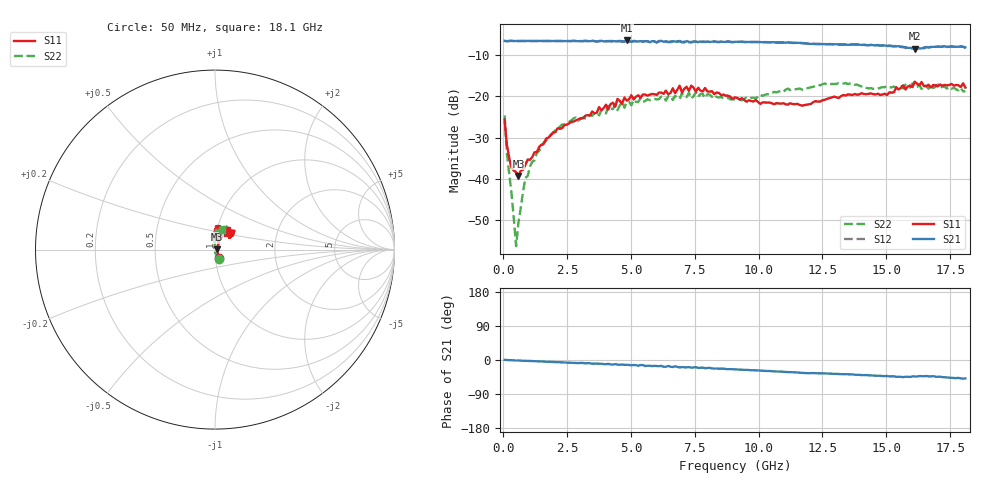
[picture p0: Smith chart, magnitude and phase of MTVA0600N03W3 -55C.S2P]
! Network Analyzer HP8720D.06.14 Serial No. US36140669
!  8 Jul 2005  09:57:14
! Frequency  S11  S21  S12  S22
# HZ  S  DB R 50
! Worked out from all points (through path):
!   201 points, 50 MHz to 18.1 GHz, reference 50 ohm
!   highest |S21| = -6.50 dB at 4.833 GHz (marker M1); lowest = -8.5 dB at 16.11 GHz (marker M2)
!   group delay of S21, straight-line fit = 7.68 ps
!   lowest |S11| = -39.2 dB at 591.5 MHz (marker M3), VSWR 1.02, Z = 51.1 + j0.0803 ohm
!   |S11| at or under -10 dB: start of sweep to end of sweep
!   |S22| runs from -56.3 to -16.8 dB; largest |S21 - S12| = 0.017
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5e7  -25.71 -67.1  -6.58 0.4  -6.62 0.3  -24.64 -67.0
1.4025e8  -31.84 -52.1  -6.69 -0.1  -6.68 -0.2  -33.88 -83.3
2.305e8  -34.84 -37.9  -6.62 -0.5  -6.62 -0.5  -38.78 -92.2
5.0125e8  -38.36 -3.4  -6.63 -1.4  -6.62 -1.3  -56.26 -169.4
5.915e8  -39.25 4.1  -6.60 -1.2  -6.65 -1.3  -50.52 133.9
8.6225e8  -36.60 26.7  -6.61 -2.0  -6.65 -2.1  -39.74 116.5
1.3135e9  -33.52 49.2  -6.61 -3.4  -6.64 -3.3  -33.73 91.3
2.30625e9  -27.70 62.6  -6.65 -6.0  -6.65 -6.1  -26.81 91.4
3.1185e9  -25.33 72.0  -6.64 -7.9  -6.68 -8.3  -25.14 98.7
4.47225e9  -20.64 69.9  -6.71 -12.1  -6.64 -11.3  -23.38 98.8
4.83325e9  -21.05 80.1  -6.50 -12.6  -6.65 -13.5  -21.39 87.6
6.09675e9  -19.10 78.1  -6.68 -16.4  -6.62 -16.4  -20.68 89.6
6.7285e9  -19.25 83.7  -6.77 -16.6  -6.95 -17.5  -19.88 84.5
6.909e9  -17.45 82.7  -6.61 -19.7  -6.74 -18.5  -20.64 82.0
6.99925e9  -19.09 82.4  -6.89 -18.5  -6.96 -19.9  -19.17 83.7
7.36025e9  -17.45 77.8  -7.01 -20.2  -6.84 -19.4  -20.54 87.9
7.54075e9  -18.89 78.6  -6.82 -19.0  -6.72 -21.0  -19.05 87.5
9.075e9  -20.26 88.5  -6.82 -24.7  -6.82 -24.8  -20.73 74.4
1.21435e10  -21.39 61.8  -7.33 -34.5  -7.29 -34.7  -17.68 64.5
1.512175e10  -19.05 39.4  -7.84 -43.3  -7.71 -43.1  -17.83 65.1
1.61145e10  -16.46 43.7  -8.49 -43.4  -8.26 -43.6  -17.84 64.1
1.81e10  -17.90 58.3  -8.18 -48.5  -8.32 -49.4  -18.80 71.5
